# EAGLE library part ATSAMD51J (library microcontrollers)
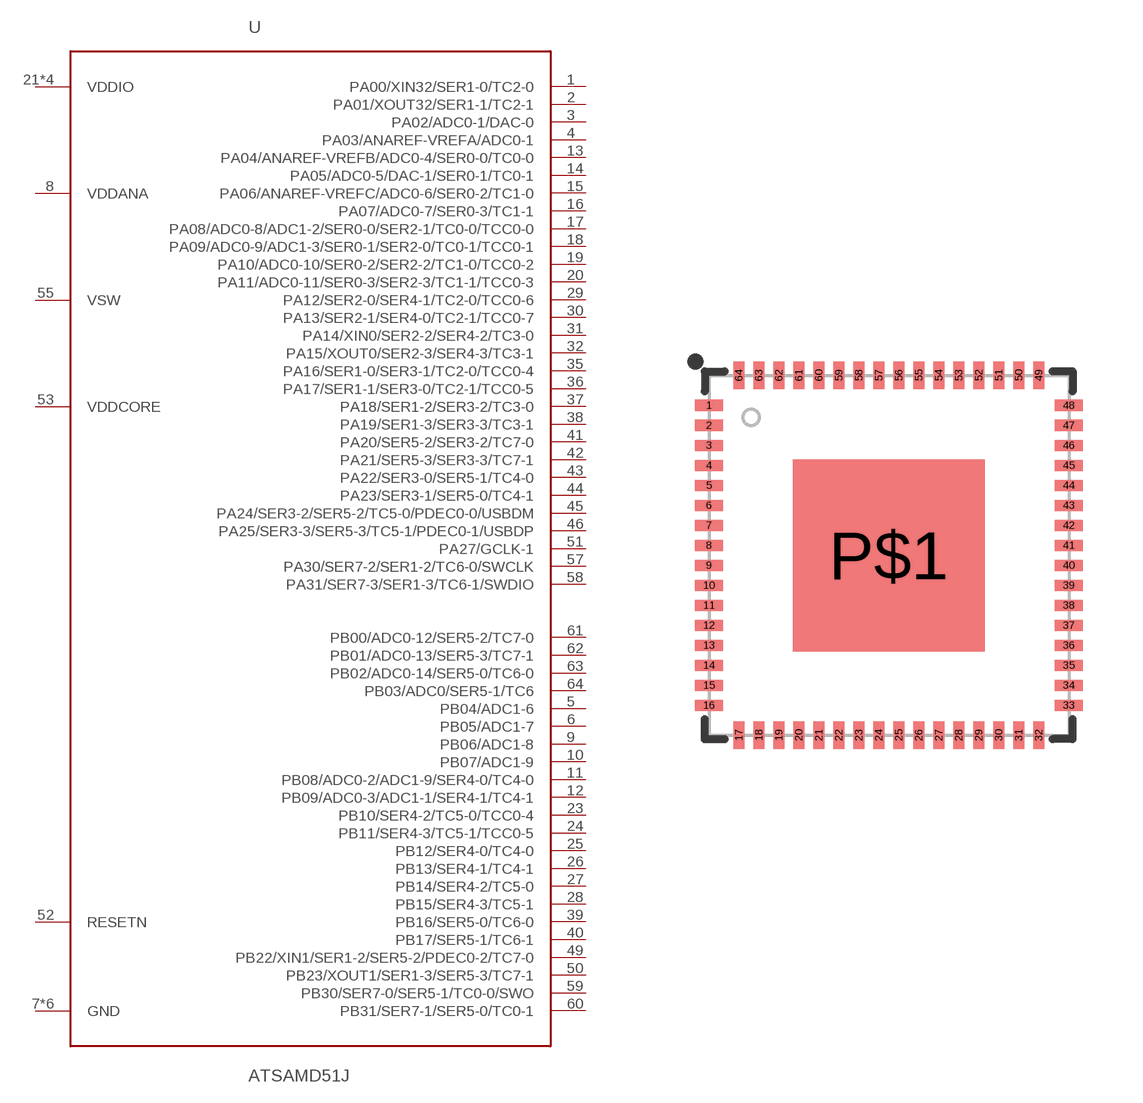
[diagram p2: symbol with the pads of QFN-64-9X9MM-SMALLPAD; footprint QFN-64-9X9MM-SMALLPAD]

Designator prefix U

## ATSAMD51JQFN64  [QFN-64-9X9MM-SMALLPAD]
1  PA00/XIN32/SER1-0/TC2-0
2  PA01/XOUT32/SER1-1/TC2-1
3  PA02/ADC0-1/DAC-0
4  PA03/ANAREF-VREFA/ADC0-1
5  PB04/ADC1-6
6  PB05/ADC1-7
7  GND
8  VDDANA
9  PB06/ADC1-8
10  PB07/ADC1-9
11  PB08/ADC0-2/ADC1-9/SER4-0/TC4-0
12  PB09/ADC0-3/ADC1-1/SER4-1/TC4-1
13  PA04/ANAREF-VREFB/ADC0-4/SER0-0/TC0-0
14  PA05/ADC0-5/DAC-1/SER0-1/TC0-1
15  PA06/ANAREF-VREFC/ADC0-6/SER0-2/TC1-0
16  PA07/ADC0-7/SER0-3/TC1-1
17  PA08/ADC0-8/ADC1-2/SER0-0/SER2-1/TC0-0/TCC0-0
18  PA09/ADC0-9/ADC1-3/SER0-1/SER2-0/TC0-1/TCC0-1
19  PA10/ADC0-10/SER0-2/SER2-2/TC1-0/TCC0-2
20  PA11/ADC0-11/SER0-3/SER2-3/TC1-1/TCC0-3
21  VDDIO
22  GND
23  PB10/SER4-2/TC5-0/TCC0-4
24  PB11/SER4-3/TC5-1/TCC0-5
25  PB12/SER4-0/TC4-0
26  PB13/SER4-1/TC4-1
27  PB14/SER4-2/TC5-0
28  PB15/SER4-3/TC5-1
29  PA12/SER2-0/SER4-1/TC2-0/TCC0-6
30  PA13/SER2-1/SER4-0/TC2-1/TCC0-7
31  PA14/XIN0/SER2-2/SER4-2/TC3-0
32  PA15/XOUT0/SER2-3/SER4-3/TC3-1
33  GND
34  VDDIO
35  PA16/SER1-0/SER3-1/TC2-0/TCC0-4
36  PA17/SER1-1/SER3-0/TC2-1/TCC0-5
37  PA18/SER1-2/SER3-2/TC3-0
38  PA19/SER1-3/SER3-3/TC3-1
39  PB16/SER5-0/TC6-0
40  PB17/SER5-1/TC6-1
41  PA20/SER5-2/SER3-2/TC7-0
42  PA21/SER5-3/SER3-3/TC7-1
43  PA22/SER3-0/SER5-1/TC4-0
44  PA23/SER3-1/SER5-0/TC4-1
45  PA24/SER3-2/SER5-2/TC5-0/PDEC0-0/USBDM
46  PA25/SER3-3/SER5-3/TC5-1/PDEC0-1/USBDP
47  GND
48  VDDIO
49  PB22/XIN1/SER1-2/SER5-2/PDEC0-2/TC7-0
50  PB23/XOUT1/SER1-3/SER5-3/TC7-1
51  PA27/GCLK-1
52  RESETN
53  VDDCORE
54  GND
55  VSW
56  VDDIO
57  PA30/SER7-2/SER1-2/TC6-0/SWCLK
58  PA31/SER7-3/SER1-3/TC6-1/SWDIO
59  PB30/SER7-0/SER5-1/TC0-0/SWO
60  PB31/SER7-1/SER5-0/TC0-1
61  PB00/ADC0-12/SER5-2/TC7-0
62  PB01/ADC0-13/SER5-3/TC7-1
63  PB02/ADC0-14/SER5-0/TC6-0
64  PB03/ADC0/SER5-1/TC6
P$1  GND

## Footprint QFN-64-9X9MM-SMALLPAD (pad centres in mm)
64-pin QFN 9x9mm, 0.5mm pitch Package used by ATmega128RFA1 Example Datasheet
smd 0.7 x 0.275: 1 -4.5,3.75; 2 -4.5,3.25; 3 -4.5,2.75; 4 -4.5,2.25; 5 -4.5,1.75; 6 -4.5,1.25; 7 -4.5,0.75; 8 -4.5,0.25; 9 -4.5,-0.25; 10 -4.5,-0.75; 11 -4.5,-1.25; 12 -4.5,-1.75; 13 -4.5,-2.25; 14 -4.5,-2.75; 15 -4.5,-3.25; 16 -4.5,-3.75; 33 4.5,-3.75; 34 4.5,-3.25; 35 4.5,-2.75; 36 4.5,-2.25; 37 4.5,-1.75; 38 4.5,-1.25; 39 4.5,-0.75; 40 4.5,-0.25; 41 4.5,0.25; 42 4.5,0.75; 43 4.5,1.25; 44 4.5,1.75; 45 4.5,2.25; 46 4.5,2.75; 47 4.5,3.25; 48 4.5,3.75
smd 0.275 x 0.7: 17 -3.75,-4.5; 18 -3.25,-4.5; 19 -2.75,-4.5; 20 -2.25,-4.5; 21 -1.75,-4.5; 22 -1.25,-4.5; 23 -0.75,-4.5; 24 -0.25,-4.5; 25 0.25,-4.5; 26 0.75,-4.5; 27 1.25,-4.5; 28 1.75,-4.5; 29 2.25,-4.5; 30 2.75,-4.5; 31 3.25,-4.5; 32 3.75,-4.5; 49 3.75,4.5; 50 3.25,4.5; 51 2.75,4.5; 52 2.25,4.5; 53 1.75,4.5; 54 1.25,4.5; 55 0.75,4.5; 56 0.25,4.5; 57 -0.25,4.5; 58 -0.75,4.5; 59 -1.25,4.5; 60 -1.75,4.5; 61 -2.25,4.5; 62 -2.75,4.5; 63 -3.25,4.5; 64 -3.75,4.5
smd 4.8 x 4.8: P$1 0,0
